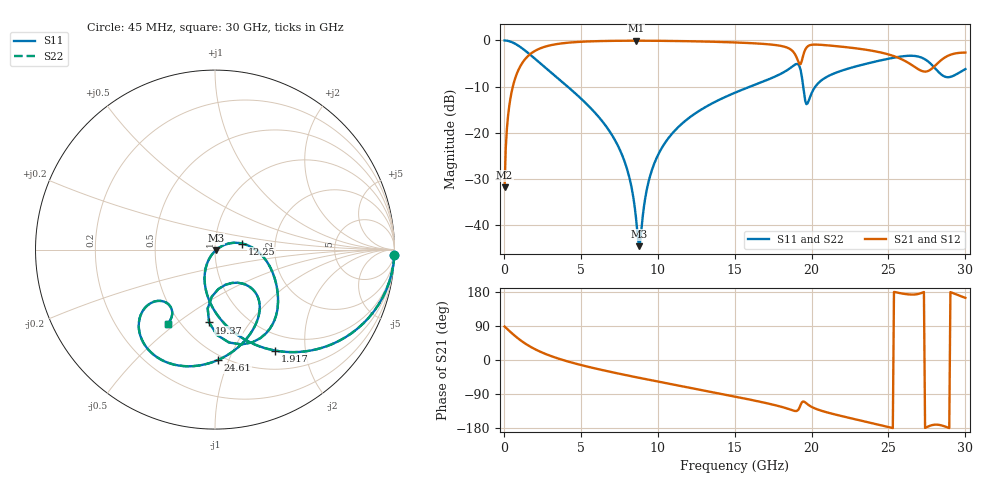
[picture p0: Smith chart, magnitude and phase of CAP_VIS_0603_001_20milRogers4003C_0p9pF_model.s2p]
! S-parameter model data by Modelithics Inc.  support@modelithics.com  813-866-6335  Tampa FL USA
! S-Parameter data specifications:
! Substrate: 20-mil Rogers 4003C, substrate thickness, H=0.508mm, Dielectric constant, Er=3.75
! PCB Mounting Pad Footprint: Pad width, PadW=0.90mm , Pad length, PadL=1.00mm , Pad gap, PadG (edge-to-edge)=1.00mm , Reference planes=3.0mm apart
! Created Wed Nov 18 13:17:16 2015
# hz S ma R 50
! 2 Port Network Data from SP1.SP block
! freq  magS11  angS11  magS21  angS21  magS12  angS12  magS22  angS22
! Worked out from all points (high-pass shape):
!   401 points, 45 MHz to 30 GHz, reference 50 ohm
!   highest |S21| = -0.06 dB at 8.582 GHz (marker M1); lowest = -31.8 dB at 45 MHz (marker M2)
!   |S21| within 3 dB of the highest: 1.673 GHz to 18.93 GHz (17.26 GHz wide, 168 % of centre); 19.47 GHz to 25.03 GHz (5.557 GHz wide, 25 % of centre)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
!   lowest |S11| = -44.5 dB at 8.807 GHz (marker M3), VSWR 1.01, Z = 50.4 - j0.411 ohm
!   |S11| at or under -10 dB: 4.144 GHz to 16 GHz (11.85 GHz wide, 118 % of centre); 19.46 GHz to 20.24 GHz (789.5 MHz wide, 3.98 % of centre)
!   |S22| runs from -44.5 to 0.0 dB; largest |S21 - S12| = 0
!   S11 on the Smith chart (normalised r, x): 45 MHz: 1, -67; 1.917 GHz: 0.75, -1.49; 12.25 GHz: 1.35, +0.09; 19.37 GHz: 0.68, -0.66; 24.61 GHz: 0.46, -0.92; 30 GHz: 0.43, -0.47
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4.5e7  0.9997 -1.7  0.02581 88.3  0.02581 88.3  0.9997 -1.7
2.696625e8  0.9882 -10.3  0.153 79.7  0.153 79.7  0.9882 -10.3
5.692125e8  0.9501 -21.2  0.3115 68.8  0.3115 68.8  0.9501 -21.2
1.917188e9  0.6554 -59.1  0.7531 30.7  0.7531 30.7  0.6554 -59.1
5.062462e9  0.2305 -102.7  0.9684 -13.8  0.9684 -13.8  0.2305 -102.7
7.53375e9  0.06578 -121.9  0.9918 -36.5  0.9918 -36.5  0.06578 -121.9
8.207738e9  0.03019 -121.4  0.9932 -42.2  0.9932 -42.2  0.03019 -121.4
8.582175e9  0.01218 -106.7  0.9934 -45.3  0.9934 -45.3  0.01218 -106.7
8.806838e9  0.005941 -43.3  0.9933 -47.1  0.9933 -47.1  0.005941 -43.3
9.405938e9  0.02972 26.0  0.9926 -52.0  0.9926 -52.0  0.02972 26.0
1.007992e10  0.06041 26.4  0.9908 -57.4  0.9908 -57.4  0.06041 26.4
1.225166e10  0.1545 12.7  0.9794 -74.5  0.9794 -74.5  0.1545 12.7
1.50225e10  0.272 -8.6  0.9512 -96.5  0.9512 -96.5  0.272 -8.6
1.854221e10  0.4929 -45.8  0.8178 -129.7  0.8178 -129.7  0.4929 -45.8
1.936598e10  0.4071 -94.6  0.6021 -112.0  0.6021 -112.0  0.4071 -94.6
1.966552e10  0.2044 -73.2  0.8352 -114.4  0.8352 -114.4  0.2044 -73.2
2.003996e10  0.2768 -47.4  0.899 -124.5  0.899 -124.5  0.2768 -47.4
2.46081e10  0.6145 -88.3  0.7339 -173.3  0.7339 -173.3  0.6145 -88.3
2.505742e10  0.6371 -93.8  0.7012 -177.6  0.7012 -177.6  0.6371 -93.8
2.737894e10  0.6242 -132.4  0.4599 -179.2  0.4599 -179.2  0.6242 -132.4
2.842736e10  0.4286 -138.2  0.613 -172.4  0.613 -172.4  0.4286 -138.2
3e10  0.4898 -122.6  0.7393 164.0  0.7393 164.0  0.4898 -122.6
